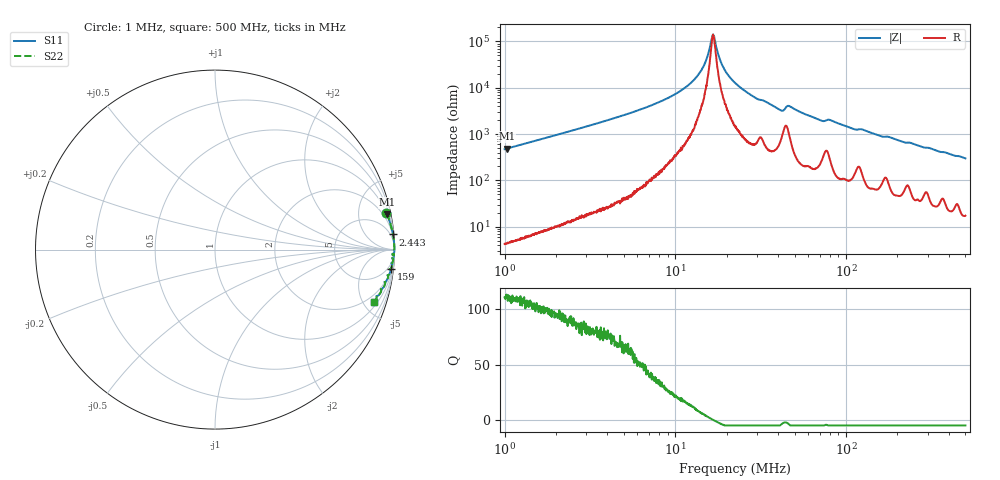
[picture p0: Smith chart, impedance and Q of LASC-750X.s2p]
!s-Parameter Generated by FASTRON Sdn. Bhd.
!FASTRON P/N : LASC-750X
!Keysight Technologies,E4991B,MY54100416,A.01.15
!Date: Tue Mar 17 15:01:16 2026
!Version  : Rev00 Tue Mar 17 15:01:16 2026
!Data & Calibration Information:
!PortZ  Port1:50+j0  Port2:50+j0
!When reading, reference impedance value at option line is always used.
! Remarks : This data is being provided solely for informational purposes.
!Freq	S11	S21	S12	S22
# Hz S dB R 50
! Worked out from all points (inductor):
!   1601 points, 1 MHz to 500 MHz, reference 50 ohm
!   read as one part in series: L = 74.8 uH near 1.032 MHz
!   highest Q = 111 at 1.032 MHz (marker M1), where L = 75.2 uH
!   self-resonance near 16.65 MHz
!   S11 on the Smith chart (normalised r, x): 1 MHz: 1.09, +9.45; 2.443 MHz: 1, +23; 159 MHz: 2, -18; 500 MHz: 1.35, -5.97
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1000000  -0.21 11.9  -13.69 -77.6  -13.69 -77.6  -0.21 11.9
1031561  -0.19 11.6  -13.95 -77.9  -13.95 -77.9  -0.19 11.6
2443301  -0.04 4.9  -21.40 -84.5  -21.40 -84.5  -0.04 4.9
2820919  -0.03 4.2  -22.70 -85.1  -22.70 -85.1  -0.03 4.2
7957584  -0.01 1.2  -33.67 -87.0  -33.67 -87.0  -0.01 1.2
1.064867e7  -0.01 0.7  -38.49 -86.2  -38.49 -86.2  -0.01 0.7
1.318477e7  -0.01 0.3  -44.29 -83.4  -44.29 -83.4  -0.01 0.3
1.487185e7  -0.01 0.2  -50.51 -77.3  -50.51 -77.3  -0.01 0.2
1.626158e7  -0.01 0.0  -60.52 -40.7  -60.52 -40.7  -0.01 0.0
1.6645e7  -0.01 0.0  -62.99 -2.2  -62.99 -2.2  -0.01 0.0
1.697142e7  -0.01 -0.0  -60.82 33.8  -60.82 33.8  -0.01 -0.0
1.805959e7  -0.01 -0.1  -53.17 70.3  -53.17 70.3  -0.01 -0.1
1.89949e7  -0.01 -0.2  -49.11 77.2  -49.11 77.2  -0.01 -0.2
2.236068e7  -0.01 -0.4  -42.08 82.8  -42.08 82.8  -0.01 -0.4
2.934708e7  -0.02 -0.9  -35.71 83.4  -35.71 83.4  -0.02 -0.9
4.098591e7  -0.05 -1.7  -30.48 77.0  -30.48 77.0  -0.05 -1.7
4.641026e7  -0.05 -1.4  -32.17 74.7  -32.17 74.7  -0.05 -1.4
6.307767e7  -0.04 -2.4  -27.53 83.2  -27.53 83.2  -0.04 -2.4
8.087875e7  -0.07 -2.8  -26.13 79.7  -26.13 79.7  -0.07 -2.8
1.589818e8  -0.13 -6.2  -19.29 79.1  -19.29 79.1  -0.13 -6.2
1.77937e8  -0.15 -6.5  -18.93 78.2  -18.93 78.2  -0.15 -6.5
5e8  -0.61 -18.1  -10.12 68.5  -10.12 68.5  -0.61 -18.1
